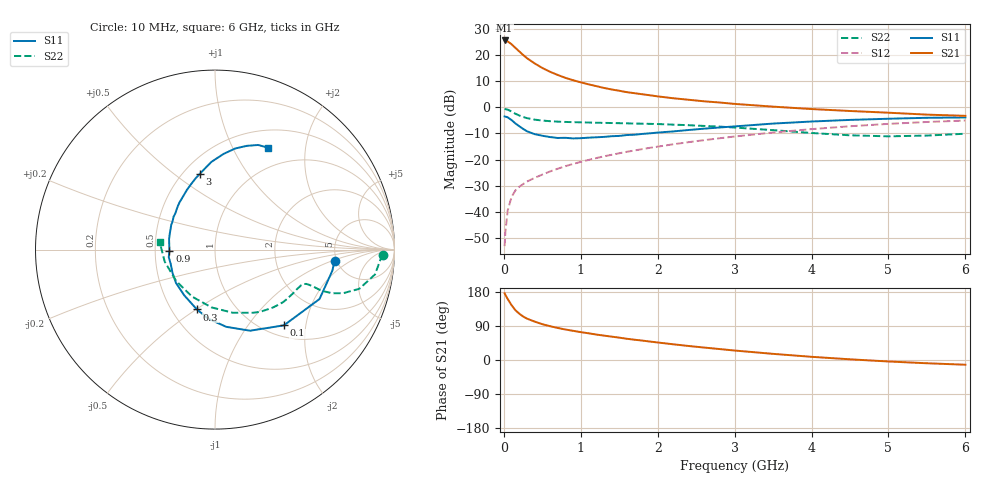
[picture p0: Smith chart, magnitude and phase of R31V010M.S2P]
! SIEMENS Small Signal Semiconductors
! BFR181
! Si NPN RF Bipolar Junction Transistor in SOT23
! VCE = 1 V  IC = 10 mA
! Common Emitter S-Parameters:  May  1996
# GHz  S  MA  R  50
!  f  S11  S21  S12  S22
! GHz  MAG  ANG  MAG  ANG  MAG  ANG  MAG  ANG
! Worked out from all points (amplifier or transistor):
!   36 points, 10 MHz to 6 GHz, reference 50 ohm
!   highest |S21| = 25.6 dB at 10 MHz (marker M1)
!   |S21| within 3 dB of that: start of sweep to 156 MHz
!   unconditionally stable (mu >= 1): 390.6 MHz to 3.962 GHz; 5.669 GHz to end of sweep
!   at 250 MHz: K = 0.79, MSG = 24.7 dB, |S12| = -29.4 dB
!   at 1.4 GHz: K = 1.27, MAG = 9.4 dB, |S12| = -18.2 dB
!   at 6 GHz: K = 1.01, MAG = 0.2 dB, |S12| = -5.1 dB
!   S11 on the Smith chart (normalised r, x): 10 MHz: 4.78, -1.09; 100 MHz: 1.21, -1.51; 300 MHz: 0.66, -0.50; 900 MHz: 0.59, -0.01; 3 GHz: 0.60, +0.63; 6 GHz: 0.72, +1.39
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0.01  0.6691 -5.4  19.06 176.0  0.0022 94.0  0.9353 -1.7
0.02  0.6643 -10.2  18.89 171.9  0.0041 86.6  0.9227 -3.6
0.05  0.6442 -25.3  18.26 160.9  0.0106 76.0  0.9024 -8.8
0.1  0.5705 -47.7  16.15 144.8  0.0192 69.8  0.8333 -15.2
0.15  0.4924 -66.6  13.74 131.4  0.0256 64.4  0.7539 -18.8
0.2  0.4349 -81.7  11.77 122.4  0.0301 61.8  0.6981 -20.4
0.25  0.3872 -95.4  10.08 114.9  0.0339 61.0  0.655 -20.9
0.3  0.3484 -106.8  8.748 109.2  0.0379 61.2  0.6213 -21.0
0.4  0.3069 -124.0  6.937 101.4  0.0446 62.3  0.5815 -20.6
0.5  0.2859 -139.5  5.669 94.5  0.0516 63.7  0.5586 -20.5
0.6  0.27 -151.2  4.796 89.2  0.0592 65.3  0.5431 -20.6
0.7  0.2591 -162.5  4.168 84.6  0.0668 66.4  0.5323 -21.1
0.9  0.2541 -178.4  3.305 77.0  0.0825 67.2  0.52 -22.3
1.1  0.2626 167.0  2.758 70.5  0.0984 68.2  0.5119 -24.5
1.3  0.2717 155.9  2.353 64.4  0.1152 67.8  0.5042 -26.9
1.6  0.2949 141.5  1.95 56.0  0.1411 67.4  0.4936 -31.2
2.2  0.3458 120.9  1.493 41.5  0.1962 64.1  0.4665 -41.6
3  0.4313 101.2  1.163 25.0  0.2763 57.1  0.41 -59.1
3.5  0.4888 92.4  1.031 16.2  0.3296 51.7  0.3659 -74.2
4.5  0.5745 78.7  0.851 1.8  0.4344 38.6  0.2914 -116.1
5.5  0.6304 67.6  0.725 -8.6  0.5243 24.1  0.288 -166.5
6  0.6408 62.3  0.687 -12.5  0.5591 16.5  0.3124 171.7
